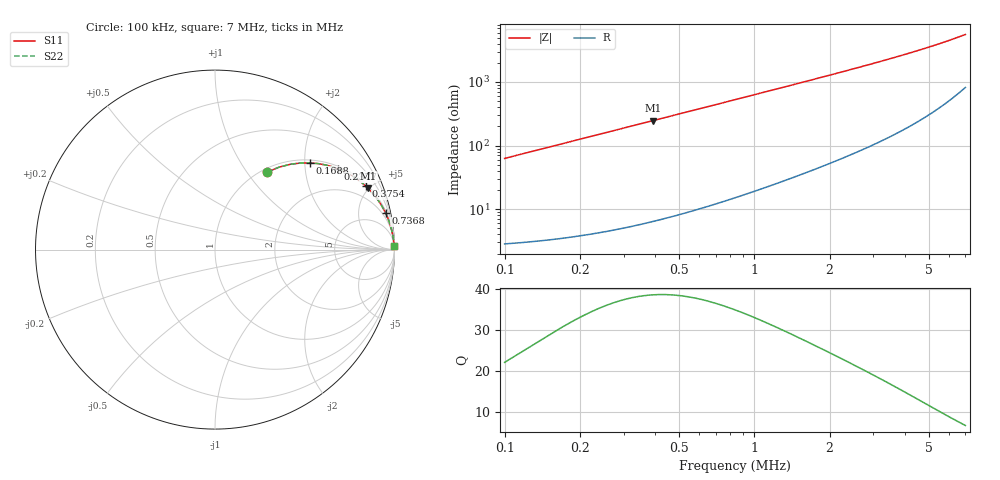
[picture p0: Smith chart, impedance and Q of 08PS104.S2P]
! Coilcraft 0805PS-104 Power Chip Inductor
! 5 February 2003
# MHZ S MA R 50
!Freq  MagS11  AngS11  MagS21  AngS21  MagS12  AngS12  MagS22  AngS22
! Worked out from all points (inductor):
!   402 points, 100 kHz to 7 MHz, reference 50 ohm
!   read as one part in series: L = 100 uH near 134.4 kHz
!   highest Q = 38.6 at 392.6 kHz (marker M1), where L = 100 uH
!   S11 on the Smith chart (normalised r, x): 100 kHz: 1.06, +1.26; 168.8 kHz: 1.07, +2.12; 237.7 kHz: 1.08, +2.99; 375.4 kHz: 1.12, +4.72; 736.8 kHz: 1.26, +9.28; 7 MHz: open
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0.1  0.5219 56.0  0.8298 -31.4  0.8298 -31.4  0.5219 56.0
0.13442  0.634 48.6  0.7502 -39.3  0.7502 -39.3  0.634 48.6
0.16884  0.7163 42.4  0.6748 -45.7  0.6748 -45.7  0.7163 42.4
0.20326  0.7763 37.4  0.6075 -50.9  0.6075 -50.9  0.7763 37.4
0.23768  0.8204 33.3  0.5491 -55.1  0.5491 -55.1  0.8204 33.3
0.2721  0.8532 29.9  0.4988 -58.5  0.4988 -58.5  0.8532 29.9
0.30652  0.8781 27.1  0.4557 -61.4  0.4557 -61.4  0.8781 27.1
0.37536  0.9123 22.7  0.3865 -65.8  0.3865 -65.8  0.9123 22.7
0.39257  0.9186 21.8  0.3721 -66.7  0.3721 -66.7  0.9186 21.8
0.46141  0.938 18.9  0.3232 -69.7  0.3232 -69.7  0.938 18.9
0.53025  0.9511 16.6  0.2851 -71.9  0.2851 -71.9  0.9511 16.6
0.73677  0.972 12.1  0.2095 -76.3  0.2095 -76.3  0.972 12.1
0.97771  0.9825 9.2  0.1592 -79.1  0.1592 -79.1  0.9825 9.2
1.25307  0.9881 7.2  0.1246 -81.0  0.1246 -81.0  0.9881 7.2
1.49401  0.9908 6.0  0.1045 -82.0  0.1045 -82.0  0.9908 6.0
1.76937  0.9928 5.0  0.08803 -82.8  0.08803 -82.8  0.9928 5.0
2.40614  0.995 3.7  0.06408 -83.7  0.06408 -83.7  0.995 3.7
2.93965  0.996 3.0  0.05179 -84.1  0.05179 -84.1  0.996 3.0
3.55921  0.9966 2.4  0.04199 -84.1  0.04199 -84.1  0.9966 2.4
4.71228  0.9971 1.7  0.03029 -83.7  0.03029 -83.7  0.9971 1.7
5.86535  0.9973 1.3  0.02291 -82.5  0.02291 -82.5  0.9973 1.3
7  0.9972 1.0  0.01781 -80.6  0.01781 -80.6  0.9972 1.0
